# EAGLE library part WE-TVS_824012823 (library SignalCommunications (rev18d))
WE-TVS TVS Diode – Super Speed Series Characteristics Operating temperature: –55 ºC to +85 °C for 824 014 x –40 ºC to +85 °C for 824 016 46 Low clamping voltage Very low capacitance Rail to Rail protection Epoxy flame resistant UL94-V0 RoHS, REACH and free of halogens Applications Super Speed data lines HDMI 1.3/1.4 DVI DisplayPort USB 3.0 SuperSpeed SATA GBit LAN Details see: http://katalog.we-online.de/en/pbs/WE-TVS-SS Created by Yingchun,Shan 2017-12-07 2017 (C) Wurth Elektronik
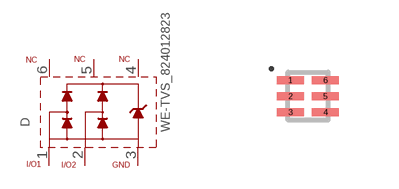
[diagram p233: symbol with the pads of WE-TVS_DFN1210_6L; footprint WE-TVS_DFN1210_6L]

Designator prefix D

## WE-TVS_824012823  [WE-TVS_DFN1210_6L]
1  I/O1
2  I/O2
3  GND
4  NC
5  NC1
6  NC2

## Footprint WE-TVS_DFN1210_6L (pad centres in mm)
smd 0.675 x 0.2: 1 -0.438,0.4; 2 -0.438,0; 3 -0.438,-0.4; 4 0.438,-0.4; 5 0.438,0; 6 0.438,0.4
